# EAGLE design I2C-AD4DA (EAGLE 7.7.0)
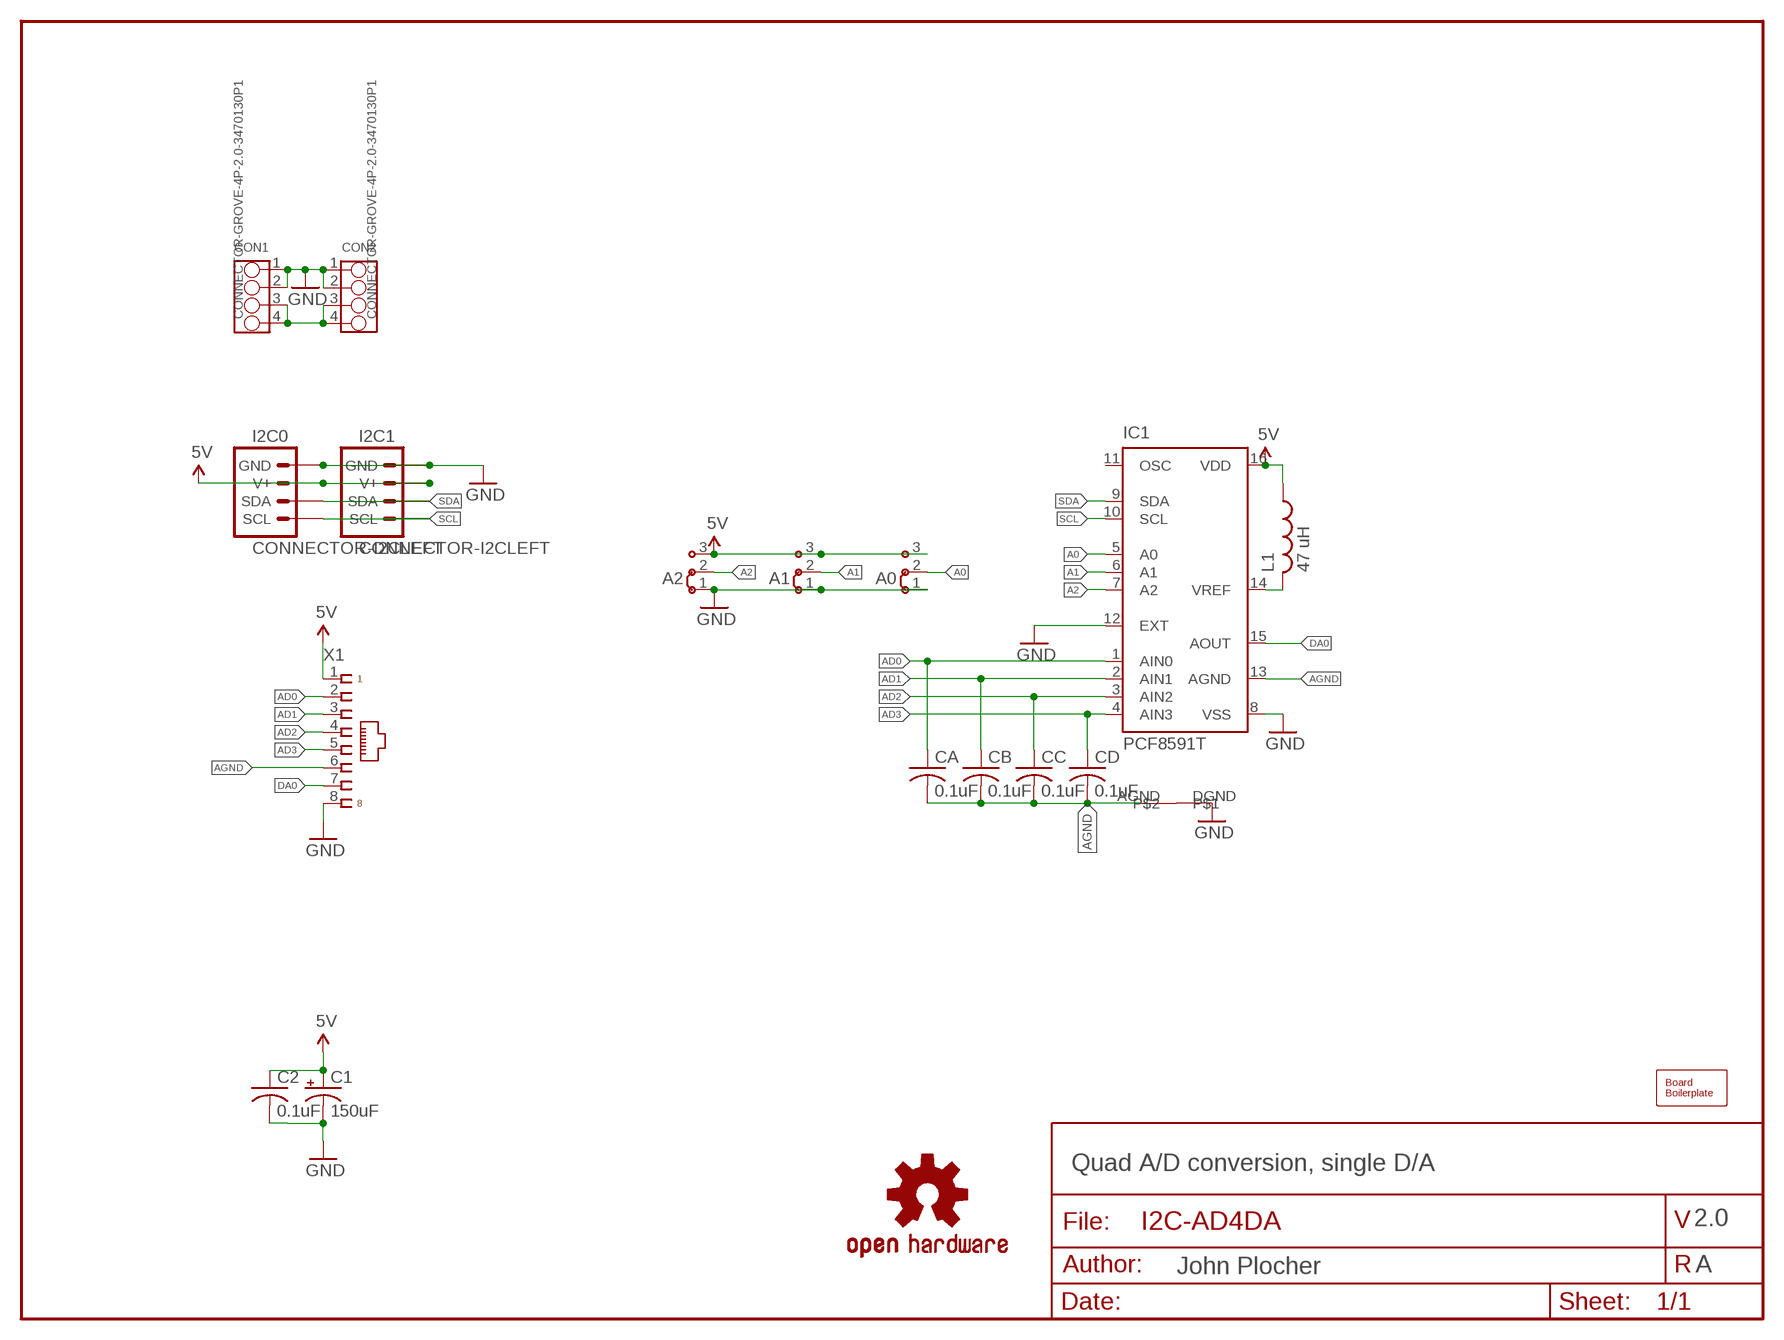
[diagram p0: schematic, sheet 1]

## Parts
A0  JUMPER-3-DEFAULT2.54MM  [J3-254]
A1  JUMPER-3-DEFAULT2.54MM  [J3-254]
A2  JUMPER-3-DEFAULT2.54MM  [J3-254]
BOARD1  BOARD80X50  [BOARD-DINRAIL-3.17INX5CM]
C1  150uF  CAP-POLUD10X10  [UD-10X10_NICHICON]
C2  0.1uF  CAP0805  [0805-CAP]
CA  0.1uF  CAP0805  [0805-CAP]
CB  0.1uF  CAP0805  [0805-CAP]
CC  0.1uF  CAP0805  [0805-CAP]
CD  0.1uF  CAP0805  [0805-CAP]
CON1  CONNECTOR-GROVE-4P-2.0-3470130P1  [4P-2.0]
CON2  CONNECTOR-GROVE-4P-2.0-3470130P1  [4P-2.0]
I2C0  CONNECTOR-I2CLEFT  [I2C-L]
I2C1  CONNECTOR-I2CLEFT  [I2C-L]
IC1  PCF8591T  [SO16W]
L1  47 uH  L-USL2012C  [L2012C]
LOGO1  DOC-OSHW-LOGO-L  [OSHW-LOGO-L]
U$1  AGND+DGND  [AGND+DGND]
X1  CONNECTOR-RJ45-FRONT  [RJ45-NO-SHIELD]

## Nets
5V: A0.3 A1.3 A2.3 C1.+ C2.1 I2C0.V+ I2C0.V+@1(V+) I2C1.V+ I2C1.V+@1(V+) IC1.16(VDD) L1.1 X1.1
A0: A0.2 IC1.5(A0)
A1: A1.2 IC1.6(A1)
A2: A2.2 IC1.7(A2)
AD0: CA.1 IC1.1(AIN0) X1.2
AD1: CB.1 IC1.2(AIN1) X1.3
AD2: CC.1 IC1.3(AIN2) X1.4
AD3: CD.1 IC1.4(AIN3) X1.5
AGND: CA.2 CB.2 CC.2 CD.2 IC1.13(AGND) U$1.AGND X1.6
DA0: IC1.15(AOUT) X1.7
GND: A0.1 A1.1 A2.1 C1.- C2.2 CON1.1 CON1.2 CON2.1 CON2.2 I2C0.GND I2C0.GND@1(GND) I2C1.GND I2C1.GND@1(GND) IC1.8(VSS) IC1.12(EXT) U$1.DGND X1.8
N$1: IC1.14(VREF) L1.2
SCL: I2C0.SCL I2C0.SCL@1(SCL) I2C1.SCL I2C1.SCL@1(SCL) IC1.10(SCL)
SDA: I2C0.SDA I2C0.SDA@1(SDA) I2C1.SDA I2C1.SDA@1(SDA) IC1.9(SDA)
VIN: CON1.3 CON1.4 CON2.3 CON2.4
Unconnected: IC1.11(OSC)

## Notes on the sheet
- Quad A/D conversion, single D/A
- 2.0
- A

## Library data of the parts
A0 A1 A2 = SPCoast:JUMPER-3-DEFAULT: Jumper switch 2 x 2.5 mm
BOARD1 = SPCoast:BOARD
C1 = SPCoast:CAP-POL*
C2 CA CB CC CD = SPCoast:CAP*
CON1 CON2 = SPCoast:CONNECTOR-GROVE-4P-2.0
I2C0 I2C1 = SPCoast:CONNECTOR-I2C
IC1 = SPCoast:PCF8591: I2C-Bus D/A CONVERTER; MPN: PCF8591T/2,512; OC_FARNELL: 1826767; OC_NEWARK: 70R6911
L1 = SPCoast:L-US: INDUCTOR, American symbol
LOGO1 = SPCoast:DOC-OSHW-LOGO-: Open Source Hardware Logo
U$1 = SPCoast:AGND+DGND
X1 = SPCoast:CONNECTOR-RJ45: Tyco CORCOM Modular RJ Jacks No Shield; AMP: 520151-4; OPL: none

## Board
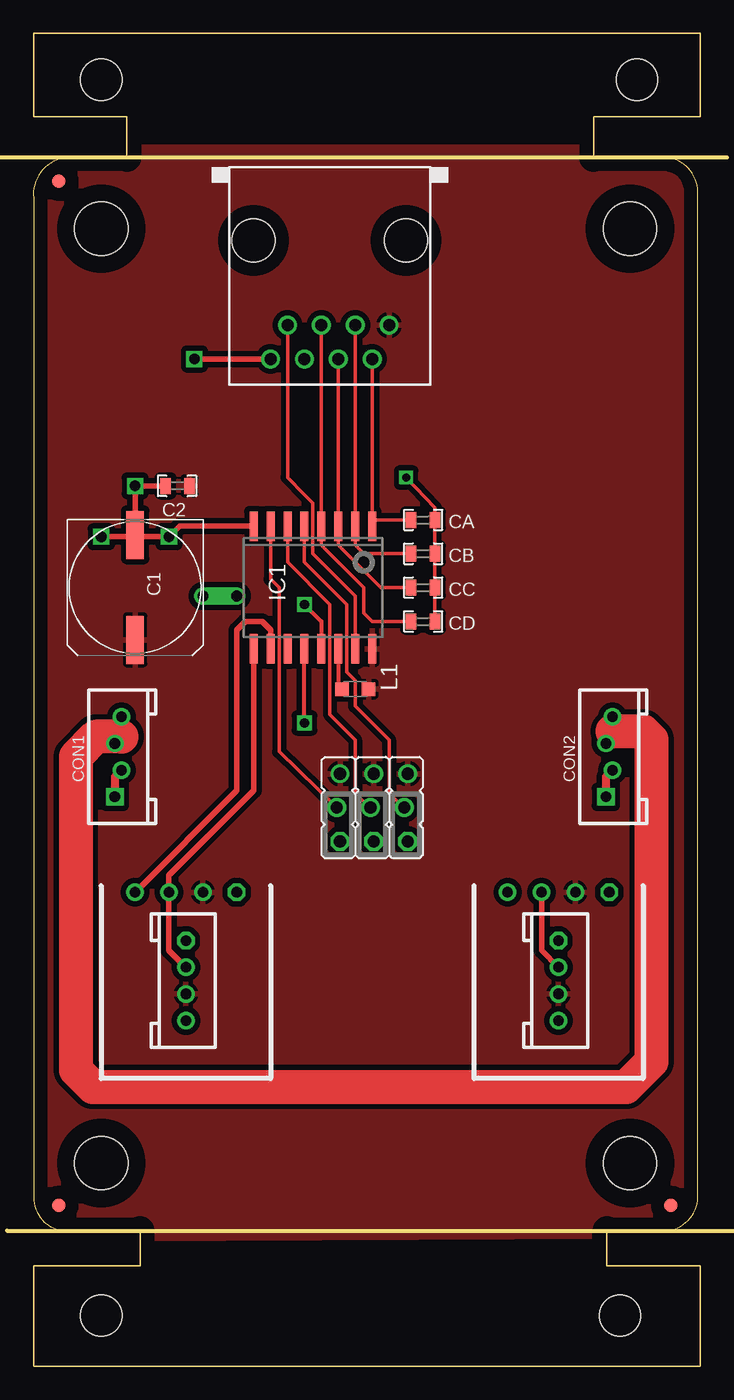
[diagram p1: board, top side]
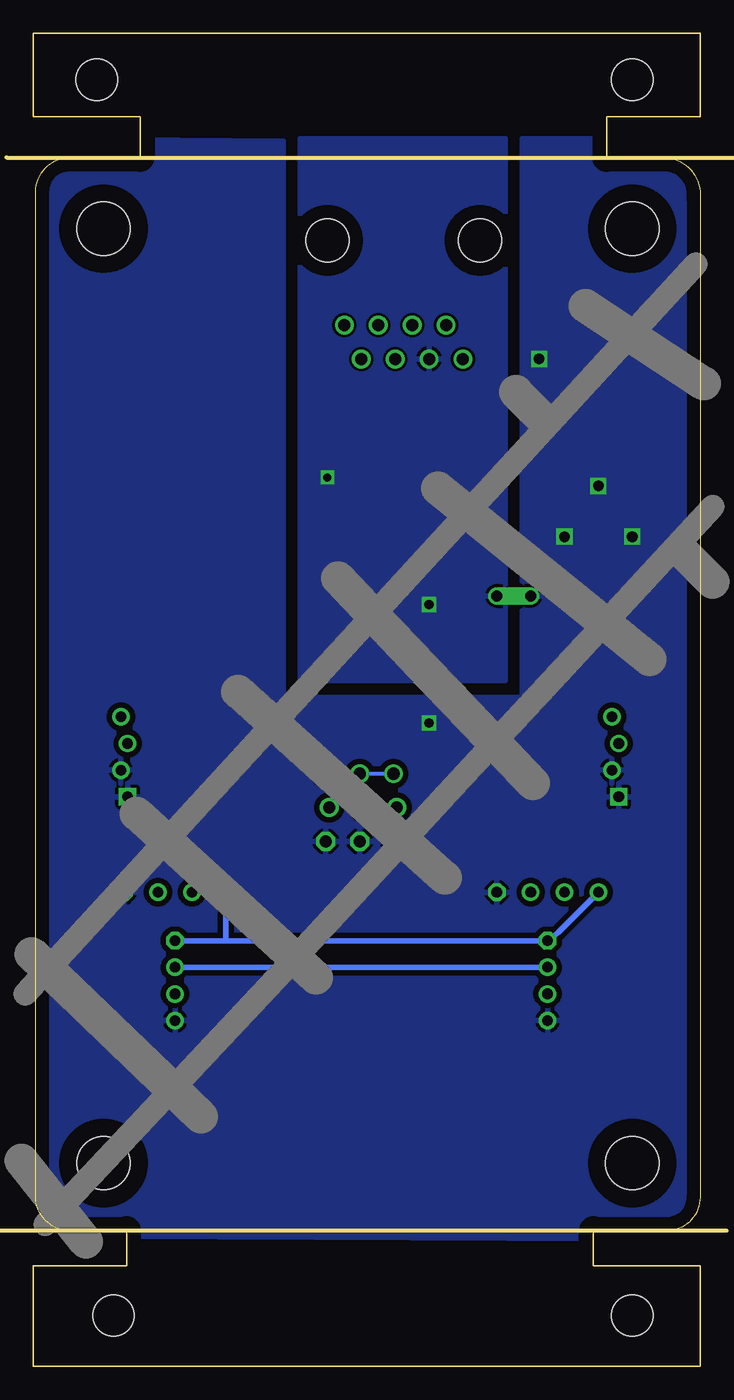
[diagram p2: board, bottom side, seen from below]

Size 50.01 x 100 mm. Coordinates in mm from the lower left corner, seen from the top.
Copper layers (1*16): Top 0.035mm / dielectric 1.5mm / Bottom 0.035mm
Design rules "default": minimum track width 10mil, minimum drill 0.6mm, track to track 8mil, track to pad 8mil, pad to pad 8mil, via to via 8mil, smd to smd 8mil, copper to edge 40mil, drill to drill 8mil, minimum pad ring 10mil, minimum via ring 8mil, stop-mask expansion 4mil, vias tented up to drill 0mil, thermal gap 10mil

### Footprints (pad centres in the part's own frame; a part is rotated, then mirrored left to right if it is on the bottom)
J3-254 = drill 0.914 octagon: 1 -2.54,-0.127 | drill 0.914: 2 0,0.127; 3 2.54,-0.127
BOARD-DINRAIL-3.17INX5CM = smd 1 x 1: 1 1.905,12.065; 2 47.79,12.065; 3 1.905,88.9 | hole 4: 44.742,15.24; 5.08,85.344; 44.742,85.344; 5.08,15.24 | hole 3.1: 5.08,96.52; 45.25,96.52; 5.08,3.81; 43.98,3.81
UD-10X10_NICHICON = smd 3.6 x 1.3: + 3.925,0; - -3.95,0
0805-CAP = smd 0.8 x 1.2: 1 -0.9,0; 2 0.9,0
4P-2.0 = drill 0.8 pad 1.27 square: 1 -3,0.254 | drill 0.8 pad 1.27: 2 -1,-0.254; 3 1,0.254; 4 3,-0.254
I2C-L = drill 0.8 octagon: GND 3.81,0 | drill 0.8 pad 1.27: GND@1 0,-9.635; SDA@1 0,-5.635; V+@1 0,-7.635 | drill 0.8: SCL -3.81,0; SDA -1.27,0; V+ 1.27,0 | drill 0.8 pad 1.27 octagon: SCL@1 0,-3.635
SO16W = smd 0.6 x 2.2: 1 -4.445,-4.6; 2 -3.175,-4.6; 3 -1.905,-4.6; 4 -0.635,-4.6; 5 0.635,-4.6; 6 1.905,-4.6; 7 3.175,-4.6; 8 4.445,-4.6; 9 4.445,4.6; 10 3.175,4.6; 11 1.905,4.6; 12 0.635,4.6; 13 -0.635,4.6; 14 -1.905,4.6; 15 -3.175,4.6; 16 -4.445,4.6
L2012C = smd 1 x 1: 1 -1,0; 2 1,0
AGND+DGND = drill 0.8 offset: AGND -1.27,0; DGND 1.27,0
RJ45-NO-SHIELD = drill 0.9 pad 1.4: 1 -4.445,6.35; 2 -3.175,8.89; 3 -1.905,6.35; 4 -0.635,8.89; 5 0.635,6.35; 6 1.905,8.89; 7 3.175,6.35; 8 4.445,8.89 | hole 3.251: -5.715,0; 5.715,0

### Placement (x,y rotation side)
A0  27.95,41.91 90 top
A1  25.41,41.91 90 top
A2  22.87,41.91 90 top
BOARD1  0.01,0 0 top
C1  7.63,58.42 270 top
C2  10.81,66.04 180 top
CA  29.22,63.5 0 top
CB  29.22,60.96 0 top
CC  29.22,58.42 0 top
CD  29.22,55.88 0 top
CON1  6.36,45.72 90 top
CON2  43.19,45.72 90 top
I2C0  11.44,35.56 0 top
I2C1  39.38,35.56 0 top
IC1  20.97,58.42 180 top
L1  24.14,50.8 180 top
LOGO1  7.63,77.47 0 top
U$1  13.98,57.78 180 top
X1  22.24,84.45 180 top

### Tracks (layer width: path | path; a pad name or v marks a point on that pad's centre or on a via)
5V
  Bottom 0.305: A2.3 A1.3 A0.3
  pour Top (isolate 0.406): 0.01,91.44 50.48,91.44 50.48,9.79 0.01,9.53
A0
  Top 0.254: IC1.5 20.33,60.33 23.51,57.15 23.51,52.07 24.14,51.44 24.14,49.53 25.41,48.26 26.68,46.99 26.68,46.35 26.68,42.93 A0.2
A1
  Top 0.254: IC1.6 19.06,60.33 22.24,57.15 22.24,48.9 24.14,46.99 24.14,42.93 A1.2
A2
  Top 0.254: IC1.7 17.79,59.05 18.43,58.42 18.43,46.1 A2.2
AD0
  Top 0.254: X1.2 25.41,71.12 25.41,69.85 25.41,63.5 | 25.41,63.5 IC1.1 25.41,63.5 | CA.1 25.41,63.5
AD1
  Top 0.254: X1.3 24.14,67.94 24.14,67.31 IC1.2 24.14,61.59 24.78,60.96 CB.1
AD2
  Top 0.254: X1.4 22.87,73.66 22.87,67.31 IC1.3 22.87,61.59 26.05,58.42 CC.1
AD3
  Top 0.254: X1.5 21.6,67.94 21.6,66.04 IC1.4 21.6,61.59 24.78,58.42 24.78,56.52 25.41,55.88 CD.1
AGND  (via drill 0.6, 0.7)
  Top 0.254: CD.2 CC.2 CB.2 CA.2 30.12,64.4 v27.95,66.67
  Top 0.305: IC1.13 21.6,55.88 v20.33,57.15
  pour Bottom: 14.62,51.44 14.62,92.08 29.99,92.08 29.99,51.44
DA0
  Top 0.254: X1.7 19.06,66.67 20.33,65.41 20.97,64.77 20.97,60.96 24.14,57.78 IC1.15
GND  (via drill 0.7, 0.8)
  Top 0.305: v20.33,48.26 IC1.12
  Top 0.406: 16.52,63.5 IC1.8 15.1,63.02 10.96,63.02 v10.17,62.23 7.63,62.23 7.63,63.5 v7.63,66.04 C2.2 | v5.09,62.23 7.49,62.23 C1.- | X1.8 v12.08,75.56
  Top 0.61: CON1.2 6.11,44.21 CON1.1 | CON2.2 42.94,44.21 CON2.1
  pour Bottom (isolate 0.406): 0.01,92.08 13.35,92.08 13.35,50.16 31.26,50.16 31.26,91.92 50.66,92.08 50.66,9.79 0.01,9.53
N$1
  Top 0.305: IC1.14 22.87,51.07 L1.2
SCL
  Top 0.406: IC1.10 17.79,55.24 17.16,55.88 15.89,55.88 15.25,55.24 15.25,43.18 I2C0.SCL
  Bottom 0.406: I2C0.SCL 10.63,32.56 I2C0.SCL@1 35.57,31.93 | 35.57,31.93 I2C1.SCL@1 | I2C1.SCL 35.57,31.93
SDA
  Top 0.406: I2C0.SDA@1 10.17,31.2 I2C0.SDA 10.17,36.83 16.52,43.18 IC1.9 | I2C1.SDA 38.11,31.2 I2C1.SDA@1
  Bottom 0.406: I2C0.SDA@1 38.11,29.93 I2C1.SDA@1
VIN
  Top 0.61: CON1.3 6.62,47.23 CON1.4 | CON2.3 43.45,47.23 43.45,47.62 CON2.4
  Top 2.54: 6.62,47.23 4.7,47.23 3.19,45.72 3.19,22.23 4.46,20.95 44.46,20.95 46.37,22.86 46.37,46.99 45.73,47.62 43.45,47.62

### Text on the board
tDocu: v2.0 | 2018-07 | OSHW | John Plocher | DA0 | AD3 | AD2 | AD1 | AD0 | +5 | I2C / 4ch A/D / 1ch D/A | Dgnd | Agnd | I2C-AD4DA | Vin | Vin | 0 1 | 5v | 5v | Board / Address | v2.0 | I2C-AD4DA
bDocu: Solder Side | Made in the PCR, Coast Division, NMRA | AD4DA | Go Bears! | Model Railroading is fun! | www . SPCoast . com | I2C / Address | A2 A1 A0 | *B0: 0 0 0 0x48 | B1: 0 0 1 0x49 | B2: 0 1 0 0x4A | B3: 0 1 1 0x4B | B4: 1 0 0 0x4C | Board / Address | B5: 1 0 1 0x4D | B6: 1 1 0 0x4E | B7: 1 1 1 0x3F

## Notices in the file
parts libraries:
SparkFun-Aesthetics: Licensing: CC v3.0 Share-Alike You are welcome to use this library for commercial purposes.
SPCoast: http://freedomdefined.org/OSHW Creative Commons - Attribution - ShareAlike 3.0
